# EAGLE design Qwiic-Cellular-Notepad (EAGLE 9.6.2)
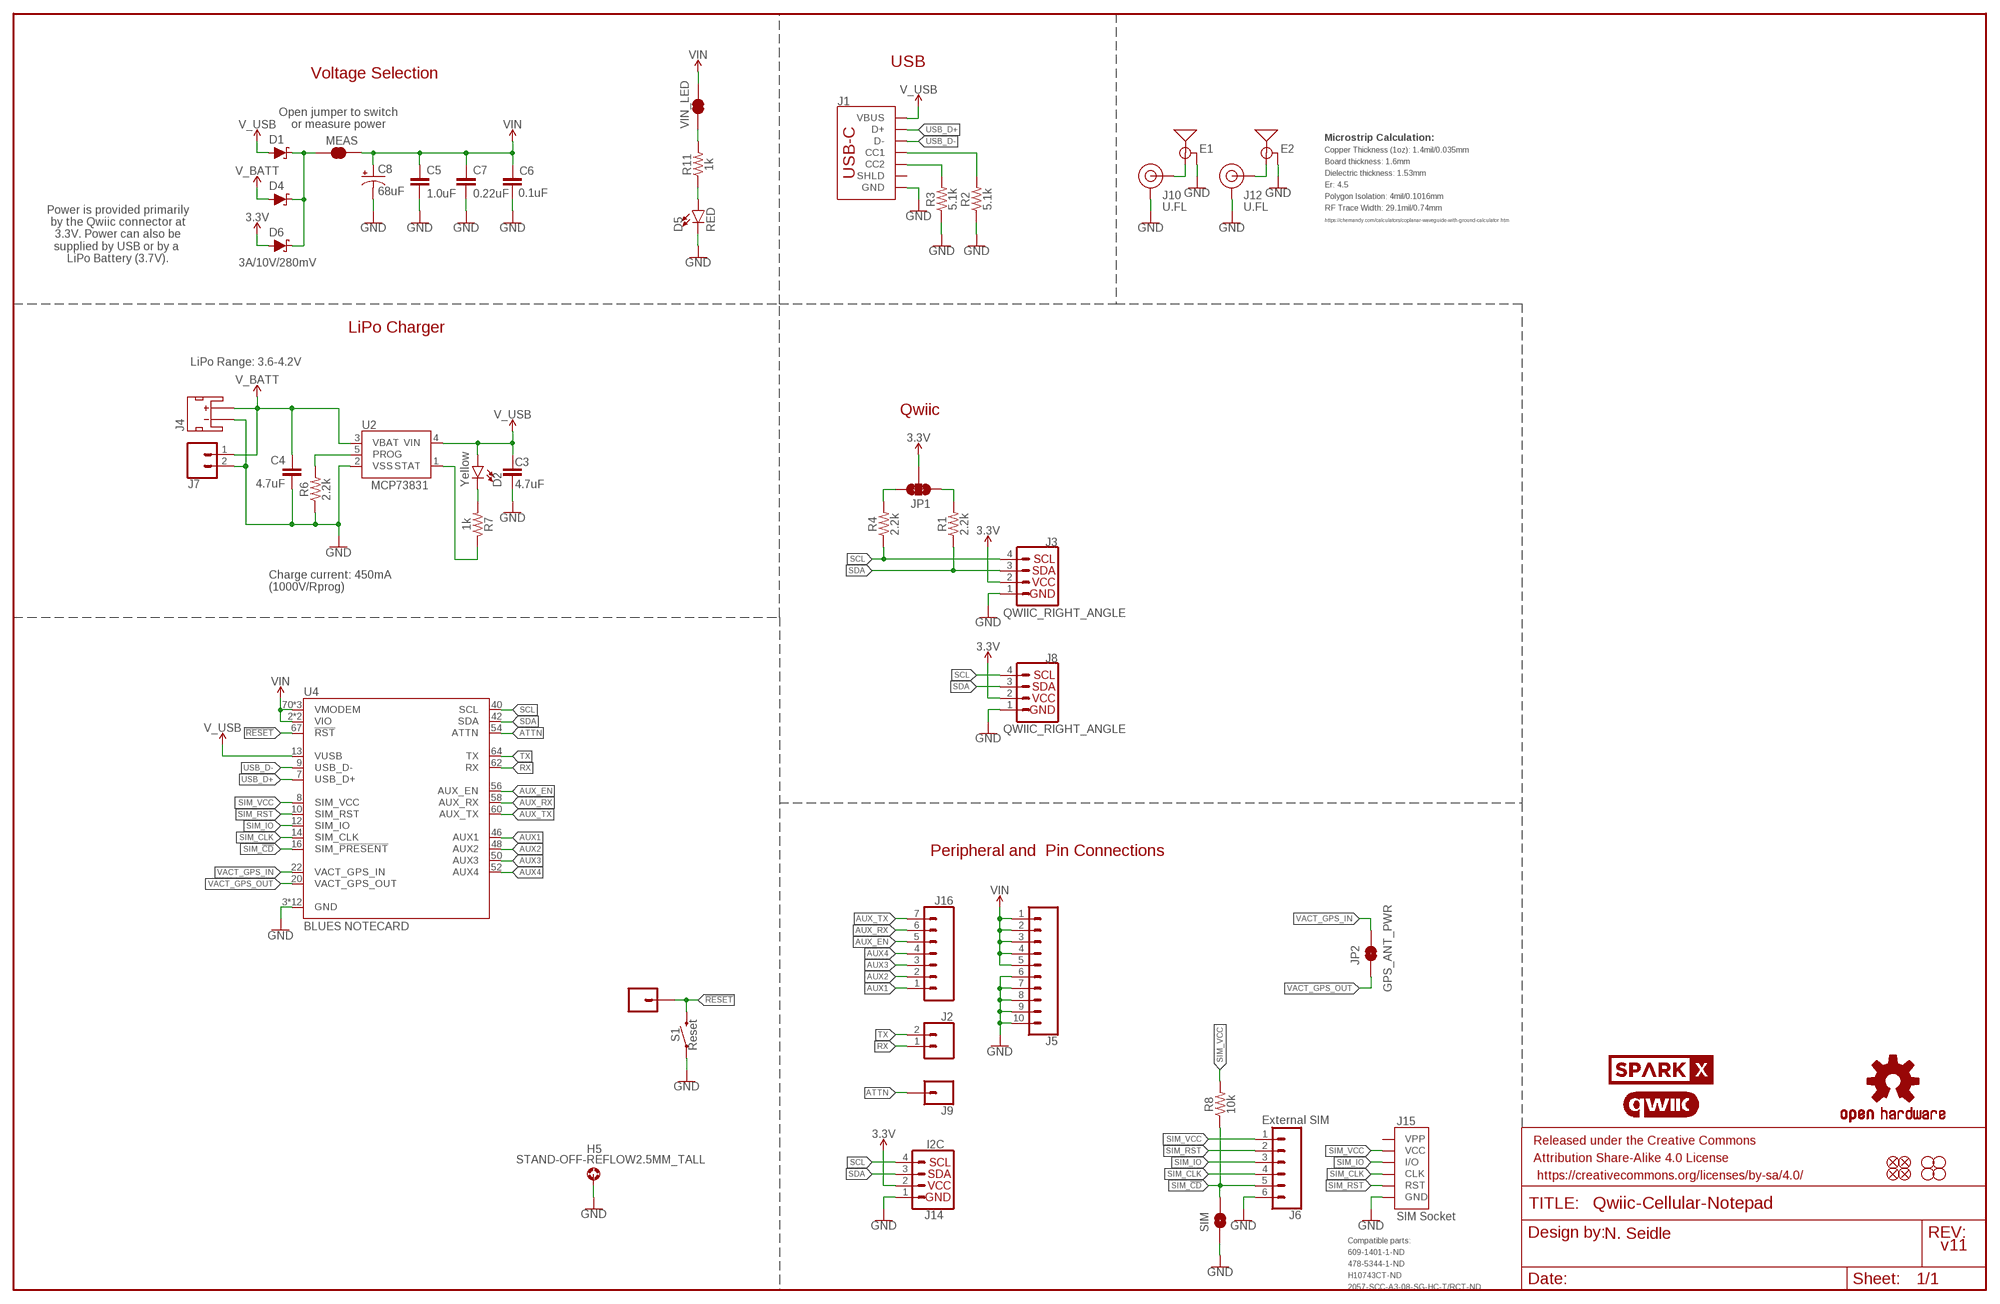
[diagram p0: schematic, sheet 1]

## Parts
C3  4.7uF  4.7UF-0603-35V-(20%)  [0603]
C4  4.7uF  4.7UF-0603-6.3V-(10%)  [0603]
C5  1.0uF  1.0UF-0603-16V-10%  [0603]
C6  0.1uF  0.1UF-0603-25V-(+80/-20%)  [0603]
C7  0.22uF  0.22UF-0603-25V-10%  [0603]
C8  68uF  68UF-POLAR-EIA3528-10V-10%(TANT)  [EIA3528]
D1  3A/10V/280mV  DIODE-SCHOTTKY-BAT60A  [SOD-323]
D2  Yellow  LED-YELLOW0603  [LED-0603]
D4  3A/10V/280mV  DIODE-SCHOTTKY-BAT60A  [SOD-323]
D5  RED  LED-RED0603  [LED-0603]
D6  3A/10V/280mV  DIODE-SCHOTTKY-BAT60A  [SOD-323]
E1  ANTENNA-GROUNDEDEDGE_SMA_SMD  [SMA-EDGE-SMD]
E2  ANTENNA-GROUNDEDEDGE_SMA_SMD  [SMA-EDGE-SMD]
FD1  FIDUCIALUFIDUCIAL  [FIDUCIAL-MICRO]
FD2  FIDUCIALUFIDUCIAL  [FIDUCIAL-MICRO]
FD3  FIDUCIALUFIDUCIAL  [FIDUCIAL-MICRO]
FD4  FIDUCIALUFIDUCIAL  [FIDUCIAL-MICRO]
FRAME1  FRAME-LEDGER  [CREATIVE_COMMONS]
H1  STAND-OFF  [STAND-OFF]
H2  STAND-OFF  [STAND-OFF]
H3  STAND-OFF  [STAND-OFF]
H4  STAND-OFF  [STAND-OFF]
H5  STAND-OFF-REFLOW2.5MM_TALL  [STAND-OFF-REFLOW-M2.5]
J1  USB_C_2-LAYER_PADS  [USB-C-16P-2LAYER-PADS]
J2  CONN_021X02_NO_SILK  [1X02_NO_SILK]
J3  QWIIC_RIGHT_ANGLE  QWIIC_CONNECTORJS-1MM  [JST04_1MM_RA]
J4  JST_2MM_MALE  [JST-2-SMD]
J5  CONN_10NO_SILK_PTH_FEMALE  [1X10_NO_SILK]
J6  External SIM  CONN_06NO_SILK_NO_POP  [1X06_NO_SILK]
J7  CONN_021X02_NO_SILK  [1X02_NO_SILK]
J8  QWIIC_RIGHT_ANGLE  QWIIC_CONNECTORJS-1MM  [JST04_1MM_RA]
J9  CONN_01PTH_NO_SILK_YES_STOP  [1X01_NO_SILK]
J10  U.FL  U.FL2PIN  [U.FL]
J12  U.FL  U.FL2PIN  [U.FL]
J13  CONN_01PTH_NO_SILK_YES_STOP  [1X01_NO_SILK]
J14  I2C  I2C_STANDARD_NO_SILK  [1X04_NO_SILK]
J15  SIM Socket  SIMHOLDERSIM  [SIMHOLDER]
J16  CONN_07NO_SILK  [1X07_NO_SILK]
JP1  JUMPER-SMT_3_2-NC_TRACE_SILK  [SMT-JUMPER_3_2-NC_TRACE_SILK]
JP2  GPS_ANT_PWR  JUMPER-SMT_2_NO_SILK  [SMT-JUMPER_2_NO_SILK]
LOGO2  QWIIC_LOGO_CONNECTOR  [QWIIC_5.5MM]
LOGO3  OSHW-LOGOMINI  [OSHW-LOGO-MINI]
MEAS  JUMPER-COMBO_2_NC_TRACE  [COMBO-JUMPER_2_NC_TRACE]
R1  2.2k  2.2KOHM-0603-1/10W-1%  [0603]
R2  5.1k  5.1KOHM5.1KOHM-0603-1/10W-1%  [0603]
R3  5.1k  5.1KOHM5.1KOHM-0603-1/10W-1%  [0603]
R4  2.2k  2.2KOHM-0603-1/10W-1%  [0603]
R6  2.2k  2.2KOHM-0603-1/10W-1%  [0603]
R7  1k  1KOHM-0603-1/10W-1%  [0603]
R8  10k  10KOHM-0603-1/10W-1%  [0603]
R11  1k  1KOHM-0603-1/10W-1%  [0603]
S1  Reset  MOMENTARY-SWITCH-SPST-SMD-5.2-TALL-REDUNDANT  [TACTILE_SWITCH_SMD_5.2MM]
SIM  JUMPER-SMT_2_NO_SILK  [SMT-JUMPER_2_NO_SILK]
U2  MCP73831  [SOT23-5]
U4  BLUES NOTECARD  NOTECARD  [M.2-CONNECTOR-E]
U$56  SPARKX-LOGO4  [SPARKX-MEDIUM]
VIN_LED  JUMPER-SMT_2_NC_TRACE_SILK  [SMT-JUMPER_2_NC_TRACE_SILK]

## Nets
3.3V: D6.A J3.2 J8.2 J14.2 JP1.2
!RESET!: J13.1 S1.3 S1.4 U4.67(!RST!)
ATTN: J9.1 U4.54(ATTN)
AUX1: J16.1 U4.46(AUX1)
AUX2: J16.2 U4.48(AUX2)
AUX3: J16.3 U4.50(AUX3)
AUX4: J16.4 U4.52(AUX4)
AUX_EN: J16.5 U4.56(AUX_EN)
AUX_RX: J16.6 U4.58(AUX_RX)
AUX_TX: J16.7 U4.60(AUX_TX)
CHG_LED: R7.1 U2.1(STAT)
GND: C3.2 C4.2 C5.2 C6.2 C7.2 C8.C(-) D5.C E1.GND@0(GND) E1.GND@1(GND) E2.GND@0(GND) E2.GND@1(GND) H5.1 J1.GND J1.GND2(GND) J3.1 J4.1(-) J5.6 J5.7 J5.8 J5.9 J5.10 J6.6 J7.2 J8.1 J10.1(GND) J10.2(GND) J12.1(GND) J12.2(GND) J14.1 J15.C5(GND) R2.1 R3.1 R6.1 S1.1 S1.2 SIM.1 U2.2(VSS) U4.3(GND) U4.5(GND) U4.6(GND) U4.11(GND) U4.18(GND) U4.33(GND) U4.39(GND) U4.45(GND) U4.51(GND) U4.57(GND) U4.71(GND) U4.73(GND)
N$2: JP1.3 R4.2
N$3: JP1.1 R1.2
N$4: D2.C R7.2
N$5: D5.A R11.1
N$6: R11.2 VIN_LED.1
N$7: R6.2 U2.5(PROG)
N$10: J1.A5(CC1) R2.2
N$11: J1.B5(CC2) R3.2
RF_GPS: E1.SIG(SIGNAL) J10.FEED(SIGNAL)
RF_LTE: E2.SIG(SIGNAL) J12.FEED(SIGNAL)
RX: J2.1 U4.62(RX)
SCL: J3.4 J8.4 J14.4 R4.1 U4.40(SCL)
SDA: J3.3 J8.3 J14.3 R1.1 U4.42(SDA)
SIM_!CD!: J6.5 R8.1 SIM.2 U4.16(SIM_!PRESENT!)
SIM_CLK: J6.4 J15.C3(CLK) U4.14(SIM_CLK)
SIM_IO: J6.3 J15.C7(I/O) U4.12(SIM_IO)
SIM_RST: J6.2 J15.C2(RST) U4.10(SIM_RST)
SIM_VCC: J6.1 J15.C1(VCC) R8.2 U4.8(SIM_VCC)
TX: J2.2 U4.64(TX)
USB_D+: J1.A6(D+) J1.B6(D+) U4.7(USB_D+)
USB_D-: J1.A7(D-) J1.B7(D-) U4.9(USB_D-)
V_BATT: C4.1 D4.A J4.2(+) J7.1 U2.3(VBAT)
V_USB: C3.1 D1.A D2.A J1.VBUS1(VBUS) J1.VBUS2(VBUS) U2.4(VIN) U4.13(VUSB)
VACT_GPS_IN: JP2.2 U4.22(VACT_GPS_IN)
VACT_GPS_OUT: JP2.1 U4.20(VACT_GPS_OUT)
VIN: C5.1 C6.1 C7.1 C8.A(+) J5.1 J5.2 J5.3 J5.4 J5.5 MEAS.2 MEAS.4 U4.2(VIO) U4.4(VIO) U4.70(VMODEM) U4.72(VMODEM) U4.74(VMODEM) VIN_LED.2
VIN1: D1.C D4.C D6.C MEAS.1 MEAS.3
Unconnected: J1.SHLD1(SHLD) J1.SHLD2(SHLD) J1.SHLD3(SHLD) J1.SHLD4(SHLD) J4.NC1(PAD1) J4.NC2(PAD2) J15.C6(VPP)

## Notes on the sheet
- USB
- Voltage Selection
- Open jumper to switch
  or measure power
- Microstrip Calculation:
- Copper Thickness (1oz): 1.4mil/0.035mm
- Board thickness: 1.6mm
- Dielectric thickness: 1.53mm
- Er: 4.5
- Polygon Isolation: 4mil/0.1016mm
- RF Trace Width: 29.1mil/0.74mm
- https://chemandy.com/calculators/coplanar-waveguide-with-ground-calculator.htm
- Power is provided primarily
  by the Qwiic connector at
  3.3V. Power can also be
  supplied by USB or by a 
  LiPo Battery (3.7V).
- LiPo Charger
- LiPo Range: 3.6-4.2V
- Qwiic
- Charge current: 450mA
  (1000V/Rprog)
- Peripheral and  Pin Connections
- N. Seidle
- Compatible parts:
- v11
- 609-1401-1-ND
- 478-5344-1-ND
- H10743CT-ND
- 2057-SCC-A3-08-SG-HC-T/RCT-ND

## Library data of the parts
C3 = SparkFun-Capacitors:4.7UF: 4.7µF ceramic capacitors; PROD_ID: CAP-14106
C4 = SparkFun-Capacitors:4.7UF: 4.7µF ceramic capacitors; PROD_ID: CAP-08280
C5 = SparkFun-Capacitors:1.0UF: 1µF ceramic capacitors; PROD_ID: CAP-00868
C6 = SparkFun-Capacitors:0.1UF: 0.1µF ceramic capacitors; PROD_ID: CAP-00810
C7 = SparkFun-Capacitors:0.22UF: 0.22µF ceramic capacitors; PROD_ID: CAP-07822
C8 = SparkFun-Capacitors:68UF-POLAR: 68µF polarized capacitors; PROD_ID: CAP-10790
D1 D4 D6 = SparkFun-DiscreteSemi:DIODE-SCHOTTKY: Schottky diode; PROD_ID: DIO-14072
D2 = SparkFun-LED:LED-YELLOW: Yellow SMD LED; PROD_ID: DIO-09003
D5 = SparkFun-LED:LED-RED: Red SMD LED; PROD_ID: DIO-00819
E1 E2 = SparkFun-RF:ANTENNA-GROUNDED: Antenna w/ Ground Connection; PROD_ID: CONN-15100
FD1-FD4 = SparkFun-Aesthetics:FIDUCIAL: Fiducial Alignment Points
FRAME1 = SparkFun-Aesthetics:FRAME-LEDGER: Schematic Frame - Ledger
H1-H4 = SparkFun-Hardware:STAND-OFF: Stand Off
H5 = SparkFun-Hardware:STAND-OFF-REFLOW: Stand Off Reflow Compatible; PROD_ID: HW-14899
J1 = SparkFun-Connectors:USB_C: USB Type C 16Pin Connector Super Speed pins not available on the 16-pin purely SMD connector so this part is best for USB 2.0 implementations. D1 and D2 are tied together enabling D+/- no matter which way the cable is plugged into the connector. The two channel configuration pins (CC1/2) are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; PROD_ID: CONN-14122
J2 J7 = SparkFun-Connectors:CONN_02: Multi connection point. Often used as Generic Header-pin footprint for 0.1 inch spaced/style header connections
J3 J8 = SparkFun-Connectors:QWIIC_CONNECTOR: SparkFun I2C Standard Qwiic Connector An SMD 1mm pitch JST connector makes it easy and quick (get it? Qwiic?) to connect I2C devices to each other. The Qwiic system enables fast and solderless connection between popular platforms and various sensors and actuators. We carry 200mm, 100mm, 50mm, and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; PROD_ID: CONN-13694
J4 = SparkFun-Connectors:JST_2MM_MALE: JST 2MM MALE RA CONNECTOR Two pin, compact surface mount connector. Commonly used as a battery input connection point. We really like the solid locking feeling and high current rating on these small connectors. We use these all the time as battery connectors. Mates to single-cell LiPo batteries.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; PROD_ID: CONN-11443; SF_ID: PRT-08612
J5 = SparkFun-Connectors:CONN_10: Multi connection point. Often used as Generic Header-pin footprint for 0.1 inch spaced/style header connections On any of the 0.1 inch spaced packages, you can populate with these: Break Away Headers - Straight (PRT-00116) Break Away Male Headers - Right Angle (PRT-00553) Female Headers (PRT-00115)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
J6 = SparkFun-Connectors:CONN_06: Multi connection point. Often used as Generic Header-pin footprint for 0.1 inch spaced/style header connections On any of the 0.1 inch spaced packages, you can populate with these: Break Away Headers - Straight (PRT-00116) Break Away Male Headers - Right Angle (PRT-00553) Female Headers (PRT-00115)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
J9 J13 = SparkFun-Connectors:CONN_01: Single connection point. Often used as Generic Header-pin footprint for 0.1 inch spaced/style header connections
J10 J12 = SparkFun-Connectors:U.FL2PIN: SMD Antenna Connector - U.FL; PROD_ID: CONN-09193; SF_ID: WRL-09144
J14 = SparkFun-Connectors:I2C_STANDARD: SparkFun I2C Standard Pinout Header SparkFun has standardized on a pinout for all I2C based sensor breakouts. This pinout allows I2C boards to be plugged directly into the headers on Arduino Uno compatible boards, and to be daisy chained easily. Example SparkFun Products: SparkFun Atmospheric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
J15 = SparkFun-Connectors:SIMHOLDER: SIM Cellular Card Socket SMT 6 pin standard connection. SparkFun Products: SIM Socket SparkFun Cellular Shield - MG2639 SparkFun SIM Card Socket Breakout; PROD_ID: CONN-08536; SF_ID: PRT-00548
J16 = SparkFun-Connectors:CONN_07: Multi connection point. Often used as Generic Header-pin footprint for 0.1 inch spaced/style header connections On any of the 0.1 inch spaced packages, you can populate with these: Break Away Headers - Straight (PRT-00116) Break Away Male Headers - Right Angle (PRT-00553) Female Headers (PRT-00115)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
JP1 = SparkFun-Jumpers:JUMPER-SMT_3_2-NC_TRACE: Normally closed trace jumper (2 of 2 connections) This jumper has a trace between all three pads so they are normally closed (NC). Use a razor knife to open the connection(s). For best results follow the IPC guidelines for cutting traces: Cutout at least 0.063 mm (0.005 in). Remove all loose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
JP2 SIM = SparkFun-Jumpers:JUMPER-SMT_2_NO: Normally open jumper
LOGO2 = SparkFun-Aesthetics:QWIIC_LOGO: Qwiic Logos for placement on schematic and PCB. The 5.5mm silk logo is best for placing next to Qwiic connector.
LOGO3 = SparkFun-Aesthetics:OSHW-LOGO: Open-Source Hardware (OSHW) Logo
MEAS = SparkFun-Jumpers:JUMPER-COMBO_2_NC_TRACE
R1 R4 R6 = SparkFun-Resistors:2.2KOHM: 2.2kΩ resistor; PROD_ID: RES-08272
R2 R3 = SparkFun-Resistors:5.1KOHM; PROD_ID: RES-12083
R7 R11 = SparkFun-Resistors:1KOHM: 1kΩ resistor; PROD_ID: RES-07856
R8 = SparkFun-Resistors:10KOHM: 10kΩ resistor; PROD_ID: RES-00824
S1 = SparkFun-Switches:MOMENTARY-SWITCH-SPST: Momentary Switch (Pushbutton) - SPST; PROD_ID: SWCH-14139
U2 = SparkFun-IC-Power:MCP73831: MCP73831T Li-Ion, Li-Pol Controller Miniature single cell, fully integrated Li-Ion, Li-polymer charge management controller Datasheet SparkFun Products: SparkFun ESP32 Thing SparkFun 9DoF Razor IMU M0; PROD_ID: IC-09995
U4 = Notecard:NOTECARD
U$56 = SparkX:SPARKX-LOGO
VIN_LED = SparkFun-Jumpers:JUMPER-SMT_2_NC_TRACE: Normally closed trace jumper

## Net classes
0 default: width 0 mm, drill 0 mm
1 power: width 0.762 mm

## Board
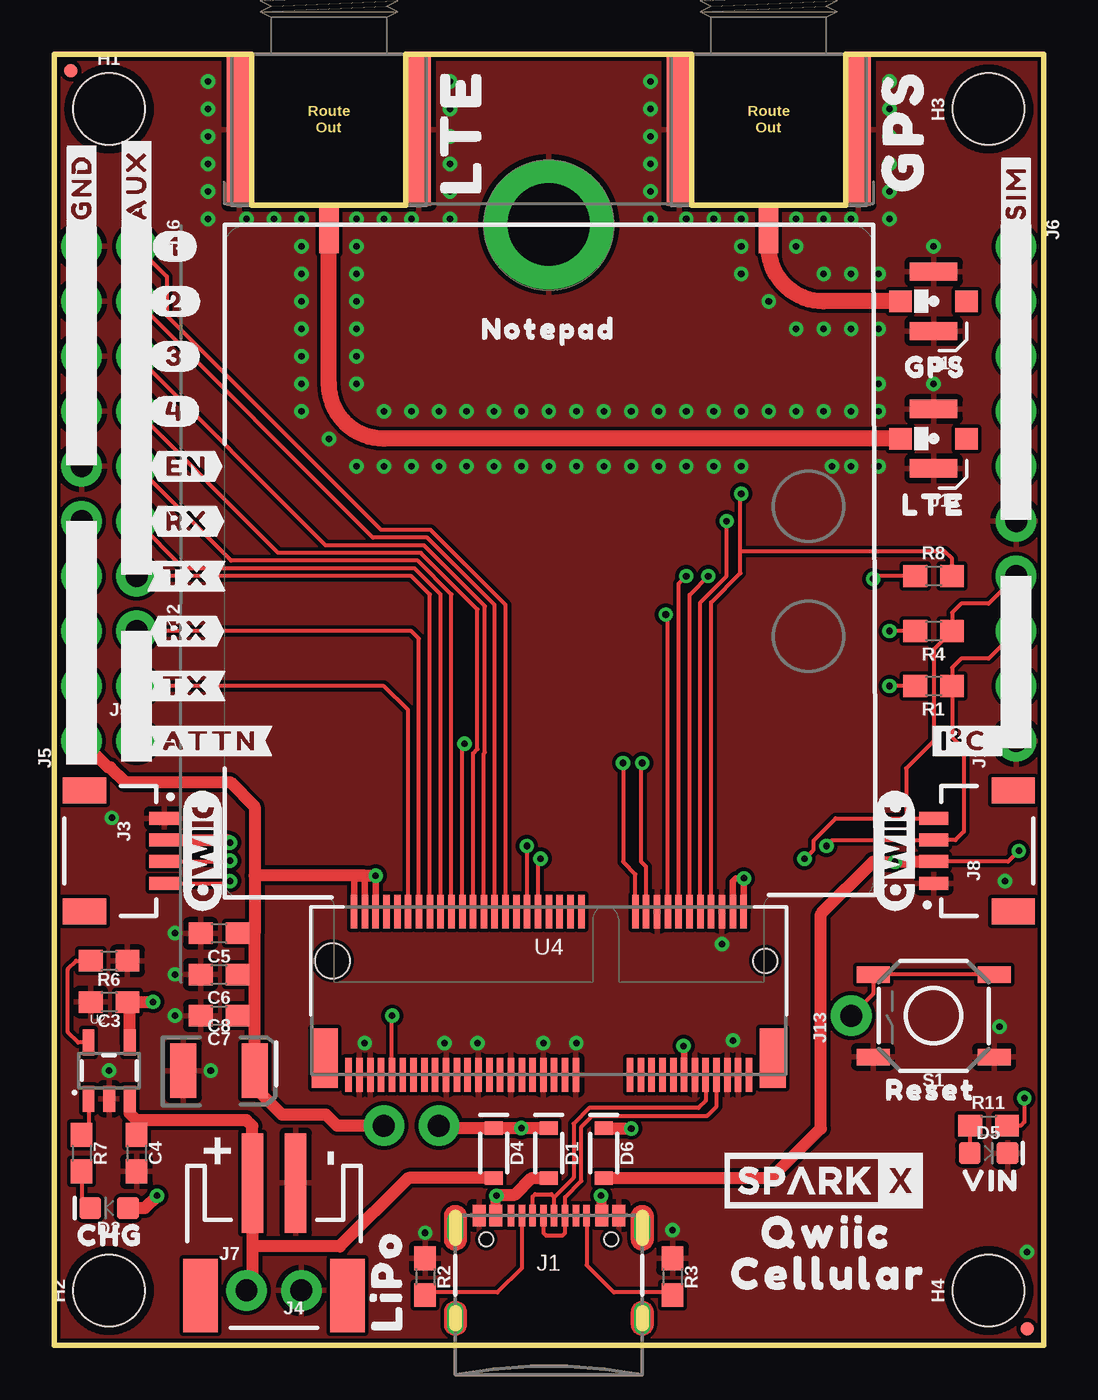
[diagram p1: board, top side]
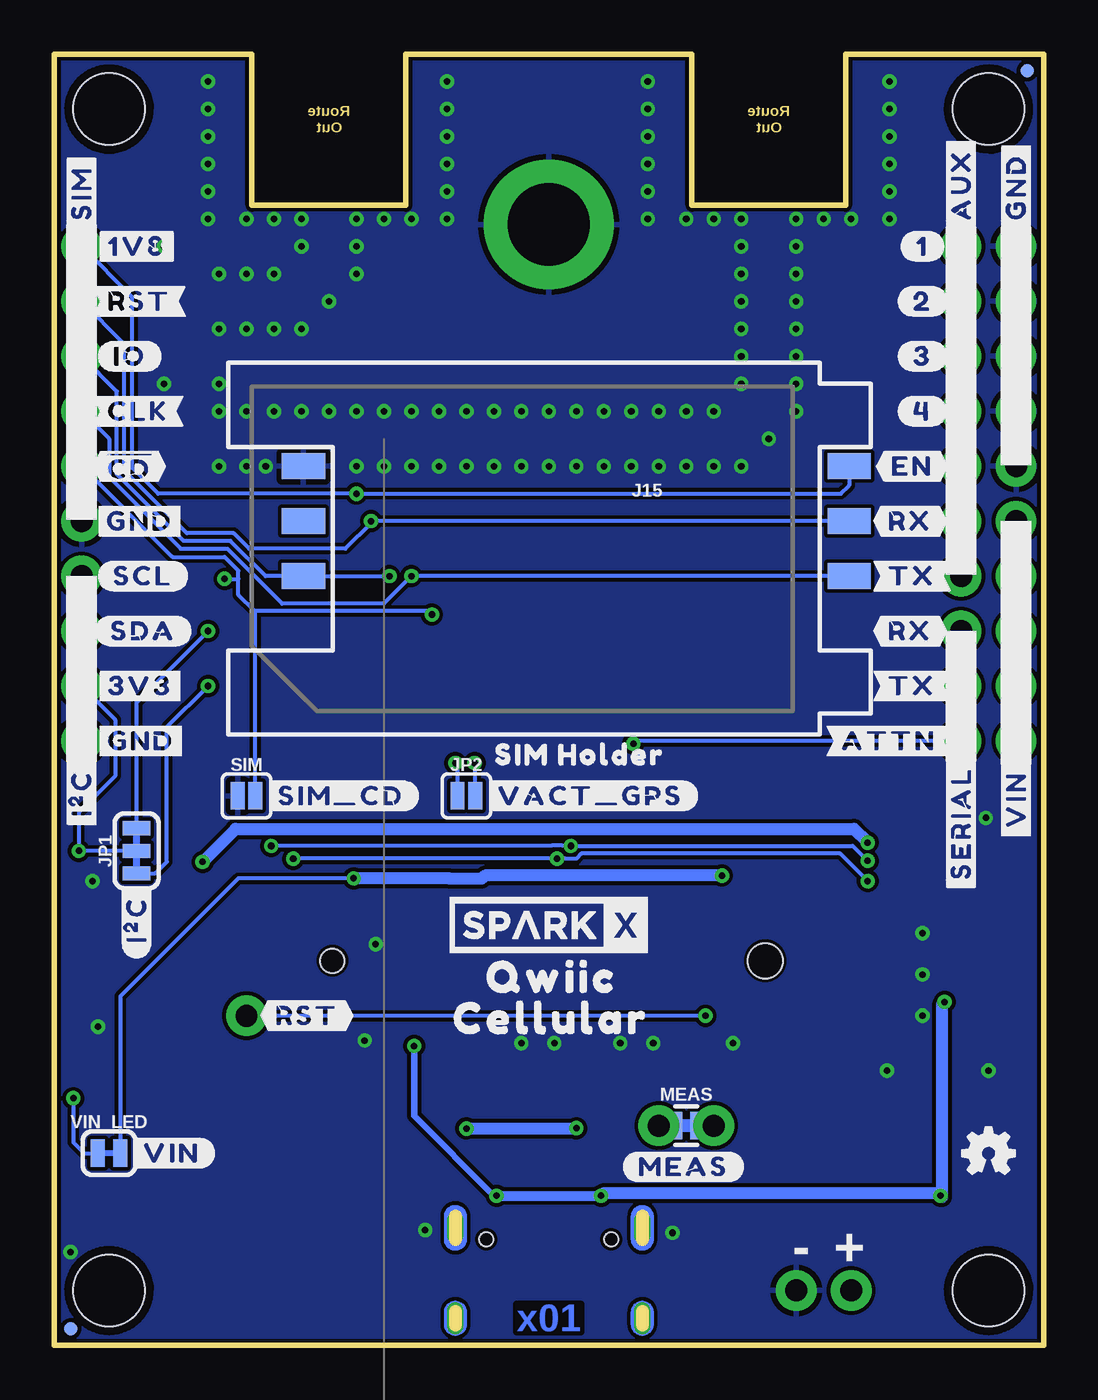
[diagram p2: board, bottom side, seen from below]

Size 45.72 x 59.69 mm. Coordinates in mm from the lower left corner, seen from the top.
Outline: 45.72,0 0,0 0,59.69 9.14,59.69 9.14,52.7 16.26,52.7 16.26,59.69 29.46,59.69 29.46,52.7 36.58,52.7 36.58,59.69 45.72,59.69 45.72,0
Copper layers (1*16): Top 0.035mm / dielectric 1.5mm / Bottom 0.035mm
Design rules "SparkFun-2-layer-TIGHT *": minimum track width 7mil, minimum drill 12mil, track to track 7mil, track to pad 7mil, pad to pad 7mil, via to via 7mil, smd to smd 7mil, copper to edge 7mil, drill to drill 7mil, minimum pad ring 7mil, minimum via ring 7mil, stop-mask expansion 4mil, vias tented up to drill 25mil, thermal gap 10mil

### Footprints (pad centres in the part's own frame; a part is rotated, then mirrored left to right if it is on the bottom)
0603 = smd 1.1 x 1: 1 -0.85,0; 2 0.85,0
EIA3528 = smd 1.2 x 2.5: A 1.65,0; C -1.65,0
SOD-323 = smd 0.63 x 0.83: A 1.15,0; C -1.15,0
LED-0603 = smd 1 x 1: A -0.877,0; C 0.877,0
SMA-EDGE-SMD = smd 1.15 x 7: GND@0 -4.14,-3.5; GND@1 4.14,-3.5 | smd 0.9 x 2.2: SIG 0,-8.1
FIDUCIAL-MICRO = smd 0.635 x 0.635: 1 0,0
STAND-OFF = hole 3.302: 0,0
STAND-OFF-REFLOW-M2.5 = drill 3.8 pad 6: 1 0,0
USB-C-16P-2LAYER-PADS = smd 0.3 x 1: A5 -1.25,-0.34; A6 -0.25,-0.34; A7 0.25,-0.34; A8 1.25,-0.34; B5 1.75,-0.34; B6 0.75,-0.34; B7 -0.75,-0.34; B8 -1.75,-0.34 | smd 0.6 x 1: GND -3.225,-0.34; GND2 3.225,-0.34; VBUS1 -2.45,-0.34; VBUS2 2.45,-0.34 | drill 0.4 pad 0.6 long: SHLD1 -4.318,-0.915; SHLD2 4.318,-0.915; SHLD3 -4.318,-5.095; SHLD4 4.318,-5.095 | hole 0.65: -2.89,-1.445; 2.89,-1.445
1X02_NO_SILK = drill 1.016 pad 1.88: 1 0,0; 2 2.54,0
JST04_1MM_RA = smd 0.6 x 1.35: 1 -1.5,0; 2 -0.5,0; 3 0.5,0; 4 1.5,0 | smd 1.2 x 2: NC1 2.8,-3.675; NC2 -2.8,-3.675
JST-2-SMD = smd 1 x 4.6: 1 -1,-3.7; 2 1,-3.7 | smd 1.6 x 3.4: NC1 -3.4,1.5; NC2 3.4,1.5
1X10_NO_SILK = drill 1.016 pad 1.88: 1 0,0; 2 2.54,0; 3 5.08,0; 4 7.62,0; 5 10.16,0; 6 12.7,0; 7 15.24,0; 8 17.78,0; 9 20.32,0; 10 22.86,0
1X06_NO_SILK = drill 1.016 pad 1.88: 1 0,0; 2 2.54,0; 3 5.08,0; 4 7.62,0; 5 10.16,0; 6 12.7,0
1X01_NO_SILK = drill 1.016 pad 1.88: 1 0,0
U.FL = smd 2.2 x 0.85: 1 0,1.375; 2 0,-1.375 | smd 1.05 x 1: FEED 1.525,0; NC -1.525,0
1X04_NO_SILK = drill 1.016 pad 1.88: 1 0,0; 2 2.54,0; 3 5.08,0; 4 7.62,0
SIMHOLDER = smd 2 x 1.2: C1 -12.61,-3.81; C2 -12.61,-1.27; C3 -12.61,1.27; C5 12.61,-3.81; C6 12.61,-1.27; C7 12.61,1.27
1X07_NO_SILK = drill 1.016 pad 1.88: 1 0,0; 2 2.54,0; 3 5.08,0; 4 7.62,0; 5 10.16,0; 6 12.7,0; 7 15.24,0
SMT-JUMPER_3_2-NC_TRACE_SILK = smd 0.66 x 1.27: 1 -1.041,0; 2 0,0; 3 1.041,0
SMT-JUMPER_2_NO_SILK = smd 0.635 x 1.27: 1 -0.406,0; 2 0.406,0
COMBO-JUMPER_2_NC_TRACE = smd 0.635 x 1.27: 1 -0.508,0; 2 0.508,0 | drill 1.016 pad 1.88: 3 -1.27,0; 4 1.27,0
TACTILE_SWITCH_SMD_5.2MM = smd 1.524 x 0.762: 1 -2.794,1.905; 2 2.794,1.905; 3 -2.794,-1.905; 4 2.794,-1.905
SOT23-5 = smd 0.55 x 1.2: 1 -0.95,-1.3; 2 0,-1.3; 3 0.95,-1.3; 4 0.95,1.3; 5 -0.95,1.3
M.2-CONNECTOR-E = smd 0.3 x 1.55: 1 9.25,-5.275; 2 9,2.275; 3 8.75,-5.275; 4 8.5,2.275; 5 8.25,-5.275; 6 8,2.275; 7 7.75,-5.275; 8 7.5,2.275; 9 7.25,-5.275; 10 7,2.275; 11 6.75,-5.275; 12 6.5,2.275; 13 6.25,-5.275; 14 6,2.275; 15 5.75,-5.275; 16 5.5,2.275; 17 5.25,-5.275; 18 5,2.275; 19 4.75,-5.275; 20 4.5,2.275; 21 4.25,-5.275; 22 4,2.275; 23 3.75,-5.275; 32 1.5,2.275; 33 1.25,-5.275; 34 1,2.275; 35 0.75,-5.275; 36 0.5,2.275; 37 0.25,-5.275; 38 0,2.275; 39 -0.25,-5.275; 40 -0.5,2.275; 41 -0.75,-5.275; 42 -1,2.275; 43 -1.25,-5.275; 44 -1.5,2.275; 45 -1.75,-5.275; 46 -2,2.275; 47 -2.25,-5.275; 48 -2.5,2.275; 49 -2.75,-5.275; 50 -3,2.275; 51 -3.25,-5.275; 52 -3.5,2.275; 53 -3.75,-5.275; 54 -4,2.275; 55 -4.25,-5.275; 56 -4.5,2.275; 57 -4.75,-5.275; 58 -5,2.275; 59 -5.25,-5.275; 60 -5.5,2.275; 61 -5.75,-5.275; 62 -6,2.275; 63 -6.25,-5.275; 64 -6.5,2.275; 65 -6.75,-5.275; 66 -7,2.275; 67 -7.25,-5.275; 68 -7.5,2.275; 69 -7.75,-5.275; 70 -8,2.275; 71 -8.25,-5.275; 72 -8.5,2.275; 73 -8.75,-5.275; 74 -9,2.275; 75 -9.25,-5.275 | smd 1.2 x 2.75: A1 10.35,-4.5; A2 -10.35,-4.5 | hole 1.1: 10,0 | hole 1.6: -10,0
SMT-JUMPER_2_NC_TRACE_SILK = smd 0.66 x 1.27: 1 -0.521,0; 2 0.521,0

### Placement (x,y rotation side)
C3  2.54,15.88 180 top
C4  3.81,8.89 270 top
C5  7.62,19.05 180 top
C6  7.62,17.14 180 top
C7  7.62,15.24 180 top
C8  7.62,12.7 0 top
D1  22.86,8.89 270 top
D2  2.54,6.35 180 top
D4  20.32,8.89 270 top
D5  43.18,8.89 0 top
D6  25.4,8.89 270 top
E1  33.02,59.69 0 top
E2  12.7,59.69 0 top
FD1  44.96,0.76 90 top
FD2  0.76,58.93 90 top
FD3  44.96,0.76 270 bottom
FD4  0.76,58.93 270 bottom
FRAME1  not placed on the board
H1  2.54,57.15 0 top
H2  2.54,2.54 90 top
H3  43.18,57.15 90 top
H4  43.18,2.54 90 top
H5  22.86,51.82 0 top
J1  22.86,6.35 0 top
J2  3.81,33.02 270 top
J3  5.08,22.86 270 top
J4  10.16,3.81 180 top
J5  1.27,27.94 90 top
J6  44.45,50.8 270 top
J7  8.89,2.54 0 top
J8  40.64,22.86 90 top
J9  3.81,27.94 0 top
J10  40.64,48.26 180 top
J12  40.64,41.91 180 top
J13  36.83,15.24 90 top
J14  44.45,27.94 90 top
J15  21.59,36.83 180 bottom
J16  3.81,50.8 270 top
JP1  41.91,22.86 90 bottom
JP2  26.67,25.4 0 bottom
LOGO2  38.86,22.86 90 top
LOGO3  2.54,8.89 0 bottom
LOGO5  QWIIC_LOGO_CONNECTOR  [QWIIC_5.5MM]  6.86,22.86 90 top
MEAS  16.51,10.16 0 bottom
R1  40.64,30.48 180 top
R2  17.14,3.17 270 top
R3  28.57,3.17 270 top
R4  40.64,33.02 180 top
R6  2.54,17.78 180 top
R7  1.27,8.89 270 top
R8  40.64,35.56 0 top
R11  43.18,10.16 0 top
S1  40.64,15.24 180 top
SIM  36.83,25.4 0 bottom
U2  2.54,12.7 0 top
U4  22.86,17.78 0 top
U$1  [#1#1]  6.6,50.8 0 bottom
U$2  [#3V3#2]  43.94,30.48 0 bottom
U$3  [#GND#0]  44.01,38.1 0 bottom
U$4  [#2#2]  6.73,48.26 0 bottom
U$5  [#3#3]  6.73,45.72 0 bottom
U$6  [#4#4]  6.73,43.18 0 bottom
U$7  [GPS_0]  39.24,51.94 90 top
U$8  [#SERIAL#1]  3.81,20.83 90 bottom
U$9  [#I�C_#0]  44.45,23.75 90 bottom
U$10  [#I�C#0]  41.91,17.91 90 bottom
U$11  [#AUX#0]  3.81,51.31 90 bottom
U$12  [LTE_1]  18.8,51.82 90 top
U$13  [#GND#3]  43.94,27.94 0 bottom
U$14  [#RX#6]  7.87,38.1 0 bottom
U$15  [LIPO0]  15.37,-0.38 90 top
U$16  [#TX#5]  7.87,35.56 0 bottom
U$17  [#SCL#1]  43.69,35.56 0 bottom
U$18  [#GND#0]  1.27,51.31 90 bottom
U$19  [#EN#0]  7.75,40.64 0 bottom
U$20  [NOTEPAD0]  19.05,46.99 0 top
U$21  [#SDA#0]  43.81,33.02 0 bottom
U$22  [#GND#0]  1.27,51.31 90 top
U$23  [#VIN#0]  1.27,23.24 90 bottom
U$24  [#VACT_GPS#0]  25.91,25.4 0 bottom
U$25  [#SIM_CD#0]  36.07,25.4 0 bottom
U$26  [QWIIC0]  26.8,17.02 0 bottom
U$27  [SIM_HOLDER0]  26.04,27.3 0 bottom
U$28  [#MEAS#3]  19.43,8.26 0 bottom
U$29  [CELLULAR1]  30.23,3.3 0 top
U$30  [#RST#0]  36.2,15.24 0 bottom
U$31  [QWIIC0]  31.62,5.21 0 top
U$32  [CELLULAR1]  28.32,15.11 0 bottom
U$33  [#VIN#1]  42.29,8.89 0 bottom
U$34  [##CD##1]  43.94,40.64 0 bottom
U$35  [#1V8#4]  43.94,50.8 0 bottom
U$36  [#CLK#3]  43.94,43.18 0 bottom
U$37  [#IO#2]  43.69,45.72 0 bottom
U$38  [#RST#5]  43.94,48.26 0 bottom
U$39  [#SIM#0]  44.45,51.31 90 bottom
U$40  [#AUX#0]  3.81,51.31 90 top
U$41  [#1#1]  4.57,50.8 0 top
U$42  [#2#2]  4.45,48.26 0 top
U$43  [#3#3]  4.45,45.72 0 top
U$44  [#4#4]  4.45,43.18 0 top
U$45  [#EN#0]  4.45,40.64 0 top
U$46  [#RX#6]  4.45,38.1 0 top
U$47  [#TX#5]  4.32,35.56 0 top
U$48  [#RX#0]  4.45,33.02 0 top
U$49  [#TX#1]  4.32,30.48 0 top
U$50  [#ATTN#2]  4.32,27.94 0 top
U$51  [#SIM#0]  44.45,51.31 90 top
U$52  [#RX#0]  7.87,33.02 0 bottom
U$53  [#I�C_#0]  40.26,27.94 0 top
U$54  [#TX#1]  7.87,30.48 0 bottom
U$55  [#ATTN#2]  10.03,27.94 0 bottom
U$56  35.56,7.62 0 top
U$57  SPARKX-LOGO4  [SPARKX-MEDIUM]  22.86,19.43 0 bottom
U$58  [GPS0]  38.61,45.21 0 top
U$59  [LTE1]  38.48,38.86 0 top
U$92  [RESET1]  37.72,11.81 0 top
U$94  [VIN1]  41.27,7.62 0 top
U$96  [CHG1]  0.38,5.08 0 top
VIN_LED  43.18,8.89 0 bottom

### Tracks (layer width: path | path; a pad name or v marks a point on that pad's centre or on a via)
3.3V  (via drill 0.3)
  Top 0.178: v44.58,22.86 44.08,22.36 J8.2
  Top 0.559: J3.2 8.01,23.36 v8.13,23.24 | J8.2 v38.87,22.36 v38.86,22.35 37.85,22.35 35.43,19.94 35.43,10.03 33.14,7.74 D6.A
  Bottom 0.178: JP1.2 v44.58,22.86 44.58,24.64 42.9,26.31 42.9,28.93 J14.2
  Bottom 0.559: v8.13,23.24 8.76,23.88 37.34,23.88 v38.86,22.35
!RESET!  (via drill 0.3)
  Top 0.178: S1.3 S1.4 37.85,16.26 J13.1 | U4.67 15.61,15.23 v15.62,15.24
  Bottom 0.178: v15.62,15.24 J13.1
ATTN  (via drill 0.3)
  Top 0.178: U4.54 18.86,27.72 v18.96,27.81
  Bottom 0.178: J9.1 18.83,27.94 v18.96,27.81
AUX1
  Top 0.178: J16.1 5.21,49.4 5.21,47.6 15.11,37.69 17.39,37.69 20.86,34.23 U4.46
AUX2
  Top 0.178: J16.2 14.73,37.34 17.25,37.34 20.36,34.22 U4.48
AUX3
  Top 0.178: J16.3 12.55,36.98 17.1,36.98 19.91,34.17 19.91,27.42 19.86,27.37 U4.50
AUX4
  Top 0.178: J16.4 10.36,36.63 16.95,36.63 19.55,34.02 19.55,27.57 19.36,27.37 U4.52
AUX_EN
  Top 0.178: U4.56 18.36,34.72 16.8,36.27 8.18,36.27 J16.5
AUX_RX
  Top 0.178: U4.58 17.86,34.71 16.66,35.92 5.99,35.92 J16.6
AUX_TX
  Top 0.178: U4.60 17.36,34.71 16.51,35.56 J16.7
CHG_LED
  Top 0.178: U2.1 1.59,10.06 R7.1
GND  (via drill 0.3)
  other vias: 2.54,12.7 7.24,12.7 5.59,15.24 5.59,17.14 5.59,19.05 2.67,24.38 43.94,21.46 43.69,14.73 31.37,14.1 19.56,13.97 22.61,13.97 24.13,13.97 18.03,13.97 14.35,13.97 30.86,18.54 17.14,5.21 28.57,5.33 44.96,4.32 27.56,58.42 27.56,57.15 27.56,55.88 27.56,54.61 27.56,53.34 27.56,52.07 35.94,40.64 29.21,52.07 30.48,52.07 31.75,52.07 34.29,52.07 35.56,52.07 36.83,52.07 38.61,52.07 38.61,53.34 38.61,54.61 38.61,55.88 38.61,57.15 38.61,58.42 18.29,58.42 18.29,57.15 18.29,55.88 18.29,54.61 18.29,53.34 18.29,52.07 16.51,52.07 15.24,52.07 13.97,52.07 11.43,52.07 10.16,52.07 8.89,52.07 7.11,52.07 7.11,53.34 7.11,54.61 7.11,55.88 7.11,57.15 7.11,58.42 11.43,50.8 11.43,49.53 11.43,48.26 11.43,46.99 11.43,45.72 11.43,44.45 11.43,43.18 12.7,41.91 13.97,40.64 15.24,40.64 16.51,40.64 17.78,40.64 19.05,40.64 20.32,40.64 21.59,40.64 22.86,40.64 24.13,40.64 25.4,40.64 26.67,40.64 27.94,40.64 29.21,40.64 30.48,40.64 31.75,40.64 36.83,40.64 38.1,40.64 13.97,44.45 15.24,43.18 16.51,43.18 17.78,43.18 19.05,43.18 20.32,43.18 21.59,43.18 22.86,43.18 24.13,43.18 25.4,43.18 26.67,43.18 27.94,43.18 29.21,43.18 30.48,43.18 31.75,43.18 13.97,50.8 13.97,49.53 13.97,48.26 13.97,46.99 13.97,45.72 33.02,43.18 34.29,43.18 35.56,43.18 36.83,43.18 38.1,43.18 40.64,44.45 38.1,44.45 31.75,50.8 31.75,49.53 33.02,48.26 34.29,46.99 35.56,46.99 36.83,46.99 38.1,46.99 38.1,49.53 36.83,49.53 35.56,49.53 34.29,50.8 40.64,50.8
  pour Bottom (isolate 0.102): 0,0 0,59.69 45.72,59.69 45.72,0
  pour Top (isolate 0.102): 0,0 0,59.69 45.72,59.69 45.72,0
N$2  (via drill 0.3)
  Top 0.178: R4.2 v38.61,33.02
  Bottom 0.178: JP1.3 41.91,29.72 v38.61,33.02
N$3  (via drill 0.3)
  Top 0.178: R1.2 v38.61,30.48
  Bottom 0.178: JP1.1 41.05,21.82 40.51,22.35 40.51,28.57 v38.61,30.48
N$4
  Top 0.178: R7.2 1.27,6.74 D2.C
N$5
  Top 0.178: R11.1 42.3,10.13 D5.A
N$6  (via drill 0.3)
  Top 0.178: v44.83,11.43 44.83,10.33 44.66,10.16 R11.2
  Bottom 0.178: v44.83,11.43 44.83,9.38 44.34,8.89 VIN_LED.1
N$7
  Top 0.178: U2.5 1.11,14 0.64,14.48 0.64,17.4 1.02,17.78 R6.2
N$10
  Top 0.178: J1.A5 21.61,3.58 20.49,2.45 17.27,2.45 R2.2
N$11
  Top 0.178: R3.2 28.45,2.45 25.87,2.45 24.61,3.71 J1.B5
RF_GPS
  Top 0.739: J10.FEED 35.56,48.26 arc-90 33.02,50.8 E1.SIG
RF_LTE
  Top 0.739: J12.FEED 15.24,41.91 arc-90 12.7,44.45 E2.SIG
RX
  Top 0.178: U4.62 16.86,32.67 16.51,33.02 J2.1
SCL  (via drill 0.3)
  Top 0.178: J3.4 8.03,21.36 v8.13,21.46 | U4.40 22.36,22.38 v22.48,22.5 | v34.67,22.49 35.09,22.91 35.09,23.34 36.11,24.36 39.37,24.36 | 39.37,24.36 J8.4 | J14.4 43.18,34.29 41.91,34.29 41.49,33.87 R4.1 40.64,32.17 40.64,27.94 39.37,26.67 39.37,24.36
  Bottom 0.178: v8.13,21.46 9.4,22.73 21.36,22.73 21.6,22.49 22.09,22.49 22.1,22.5 v22.48,22.5 34.66,22.5 v34.67,22.49
SDA  (via drill 0.3)
  Top 0.178: J3.3 8.09,22.36 v8.13,22.4 | U4.42 21.86,23.07 v21.84,23.09 | v35.69,23.09 35.96,23.36 J8.3 41.65,23.36 42.04,23.75 42.04,27.56 41.49,28.11 R1.1 41.49,31.33 41.91,31.75 43.18,31.75 J14.3
  Bottom 0.178: v8.13,22.4 8.37,22.64 8.38,22.64 8.82,23.09 v21.84,23.09 22.22,23.09 22.23,23.1 22.73,23.1 22.74,23.09 v35.69,23.09
SIM_!CD!  (via drill 0.3)
  Top 0.178: U4.16 28.36,33.69 v28.26,33.78 | R8.1 37.97,35.56 v37.85,35.43
  Bottom 0.178: v28.26,33.78 28.42,33.93 36.45,33.93 | J6.5 40.26,36.45 37.85,36.45 37.21,35.81 37.21,35.43 | v37.85,35.43 37.21,35.43 | 36.45,33.93 36.42,33.91 SIM.2 | 36.45,33.93 37.21,34.69 37.21,35.43
SIM_CLK  (via drill 0.3)
  Top 0.178: U4.14 28.86,35.21 v29.21,35.56
  Bottom 0.178: J15.C3 v29.21,35.56 30.48,34.29 35.18,34.29 37.72,36.83 39.88,36.83 43.18,40.13 43.18,41.91 J6.4
SIM_IO  (via drill 0.3)
  Top 0.178: U4.12 29.36,34.69 v30.23,35.56
  Bottom 0.178: v30.23,35.56 31.62,35.56 J15.C7 35.95,35.56 37.57,37.19 39.73,37.19 42.82,40.28 42.82,44.09 J6.3
SIM_RST  (via drill 0.3)
  Top 0.178: U4.10 29.86,34.35 31.08,35.57 v31.08,38.1
  Bottom 0.178: J15.C2 v31.08,38.1 31.08,38.01 32.26,36.83 36.71,36.83 37.42,37.54 39.58,37.54 42.47,40.43 42.47,46.28 J6.2
SIM_VCC  (via drill 0.3)
  Top 0.178: U4.8 30.36,34.35 31.71,35.7 31.71,36.7 | v31.75,39.37 31.71,39.33 31.71,36.7 | R8.2 41.49,36.36 41.15,36.7 31.71,36.7
  Bottom 0.178: J15.C1 8.98,39.75 9.36,39.37 v31.75,39.37 40.91,39.37 42.11,40.57 42.11,48.46 J6.1
TX
  Top 0.178: U4.64 16.36,29.36 15.24,30.48 J2.2
USB_D+
  Top 0.178: J1.A6 22.61,5.2 22.73,5.08 23.5,5.08 23.61,5.2 J1.B6 23.61,6.85 24.36,7.6 24.36,10.11 24.88,10.62 30.18,10.62 30.61,11.05 U4.7
USB_D-
  Top 0.178: J1.A7 23.11,6.85 | U4.9 30.11,11.31 29.77,10.98 24.73,10.98 24,10.25 24,7.75 23.11,6.85 | J1.B7 22.11,6.87 22.23,6.99 22.98,6.99 23.11,6.85
V_BATT
  Top 0.559: D4.A 16.38,7.74 13.21,4.57 9.16,4.57 | 9.16,4.57 J4.2 9.16,10.14 8.89,10.41 3.81,10.41 | 9.16,4.57 9.16,2.81 J7.1 | C4.1 3.81,10.41 | U2.3 3.49,10.73 3.81,10.41
V_USB  (via drill 0.3)
  Top 0.178: 29.11,13.82 v29.08,13.84 | 3.49,15.78 C3.1
  Top 0.305: U4.13 29.11,13.82
  Top 0.457: J1.VBUS2 25.31,6.92 v25.27,6.92 | J1.VBUS1 20.41,6.88 v20.45,6.92
  Top 0.559: v20.45,6.92 20.5,6.97 21.3,6.97 22.08,7.74 D1.A | C3.1 v4.57,15.88 | D2.A 4.19,6.35 v4.76,6.92 | U2.4 3.49,15.78
  Bottom 0.305: v29.08,13.84 29.08,10.6 25.4,6.92 v25.27,6.92
  Bottom 0.457: v25.27,6.92 v20.45,6.92
  Bottom 0.559: v20.45,6.92 20.32,7.04 4.88,7.04 v4.76,6.92 4.7,6.86 4.7,15.75 v4.57,15.88
VACT_GPS_IN  (via drill 0.3)
  Top 0.178: U4.22 26.86,21.78 26.29,22.35 v26.29,26.92
  Bottom 0.178: JP2.2 26.26,26.9 v26.29,26.92
VACT_GPS_OUT  (via drill 0.3)
  Top 0.178: U4.20 27.36,22.12 27.13,22.36 27.13,26.87 v27.18,26.92
  Bottom 0.178: JP2.1 27.08,26.82 v27.18,26.92
VIN  (via drill 0.3)
  Top 0.305: U4.74 13.86,21.61 13.97,21.72 | U4.72 14.36,21.71 14.35,21.72 | U4.70 v14.86,21.72 | U4.2 31.86,21.57 v31.88,21.59 31.5,21.59 31.36,21.45 U4.4
  Top 0.559: MEAS.4 13.08,10.16 12.57,10.67 10.54,10.67 9.27,11.94 C8.A 9.27,15.24 | 9.27,15.24 9.27,17.14 | 9.27,17.14 9.27,19.05 | C5.1 9.27,19.05 | C6.1 9.27,17.14 | C7.1 9.27,15.24 | J5.5 J5.4 J5.3 J5.2 J5.1 2.49,26.72 2.59,26.72 3.28,26.04 8.13,26.04 9.27,24.89 9.27,21.72 | 9.27,21.72 9.27,19.05 | 14.35,21.72 13.97,21.72 | 13.97,21.72 9.27,21.72 | 13.97,21.72 v14.86,21.72
  Bottom 0.178: v31.88,21.59 37.21,21.59 42.66,16.14 VIN_LED.2 | MEAS.4 MEAS.2
  Bottom 0.559: v14.86,21.72 25.81,21.72 25.96,21.57 27.45,21.57 27.47,21.59 v31.88,21.59
VIN1  (via drill 0.3)
  Top 0.559: MEAS.3 17.9,10.04 D4.C v21.59,10.04 D1.C | D6.C 26.66,10.04 v26.67,10.03
  Bottom 0.178: MEAS.1 MEAS.3
  Bottom 0.559: v26.67,10.03 21.61,10.03 v21.59,10.04

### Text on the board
Bottom: x01
tPlace: + | -
bPlace: + | -
tDocu: N. Seidle

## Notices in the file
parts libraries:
SparkFun-Aesthetics: Licensing: Creative Commons ShareAlike 4.0 International - https://creativecommons.org/licenses/by-sa/4.0
SparkFun-Aesthetics: Released under the Creative Commons Attribution Share-Alike 4.0 License
SparkFun-Aesthetics: https://creativecommons.org/licenses/by-sa/4.0
